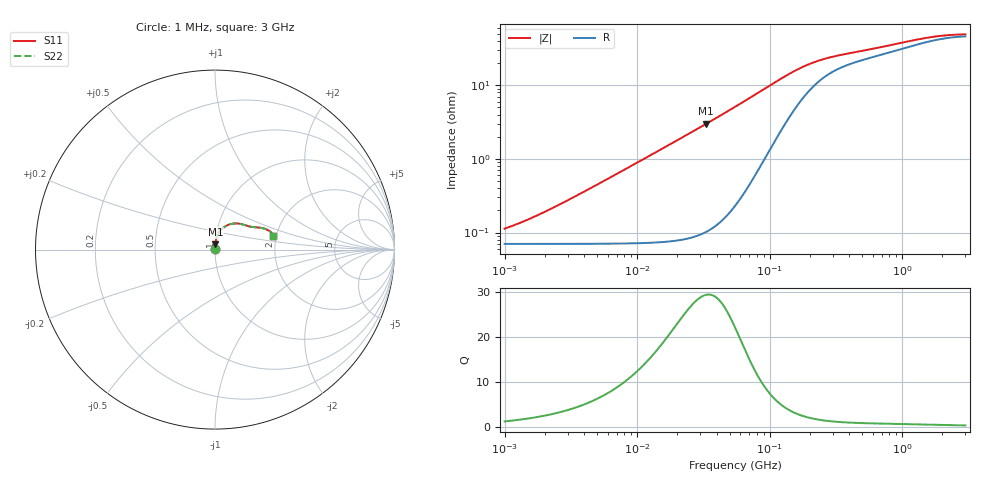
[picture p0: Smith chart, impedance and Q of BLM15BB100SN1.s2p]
! BLM15BB100SN1
# Hz S RI R 50
!Freq.(Hz) S11(Real) S11(Imag) S21(Real) S21(Imag) S12(Real) S12(Imag) S22(Real) S22(Imag)
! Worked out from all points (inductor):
!   401 points, 1 MHz to 3 GHz, reference 50 ohm
!   read as one part in series: L = 14.1 nH near 2.413 MHz
!   highest Q = 29.4 at 33.21 MHz (marker M1), where L = 14.4 nH
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1000000  0.0007 0.000884  0.9993 -0.000884  0.9993 -0.000884  0.0007 0.000884
1061887  0.000701 0.000938  0.9993 -0.000938  0.9993 -0.000938  0.000701 0.000938
1271492  0.000701 0.00112  0.9993 -0.00112  0.9993 -0.00112  0.000701 0.00112
1751453  0.000702 0.00155  0.9993 -0.00155  0.9993 -0.00155  0.000702 0.00155
2461366  0.000705 0.00217  0.9993 -0.00217  0.9993 -0.00217  0.000705 0.00217
3823119  0.000713 0.00338  0.9993 -0.00338  0.9993 -0.00338  0.000713 0.00338
1.461624e7  0.000904 0.013  0.9991 -0.013  0.9991 -0.013  0.000904 0.013
3.320783e7  0.00191 0.0299  0.9981 -0.0299  0.9981 -0.0299  0.00191 0.0299
5.477226e7  0.00485 0.0504  0.9952 -0.0504  0.9952 -0.0504  0.00485 0.0504
9.034013e7  0.0169 0.0856  0.9831 -0.0856  0.9831 -0.0856  0.0169 0.0856
1.295243e8  0.043 0.1191  0.957 -0.1191  0.957 -0.1191  0.043 0.1191
1.646891e8  0.0731 0.1376  0.9269 -0.1376  0.9269 -0.1376  0.0731 0.1376
1.857042e8  0.0908 0.1431  0.9092 -0.1431  0.9092 -0.1431  0.0908 0.1431
2.094008e8  0.1088 0.1455  0.8912 -0.1455  0.8912 -0.1455  0.1088 0.1455
2.457655e8  0.1316 0.1447  0.8684 -0.1447  0.8684 -0.1447  0.1316 0.1447
3.002264e8  0.1559 0.1397  0.8441 -0.1397  0.8441 -0.1397  0.1559 0.1397
4.66327e8  0.1951 0.1282  0.8049 -0.1282  0.8049 -0.1282  0.1951 0.1282
8.005644e8  0.2384 0.1236  0.7616 -0.1236  0.7616 -0.1236  0.2384 0.1236
1.218836e9  0.2763 0.1165  0.7237 -0.1165  0.7237 -0.1165  0.2763 0.1165
1.645649e9  0.3007 0.1052  0.6993 -0.1052  0.6993 -0.1052  0.3007 0.1052
2.221924e9  0.3176 0.0905  0.6824 -0.0905  0.6824 -0.0905  0.3176 0.0905
3e9  0.3242 0.0772  0.6758 -0.0772  0.6758 -0.0772  0.3242 0.0772
